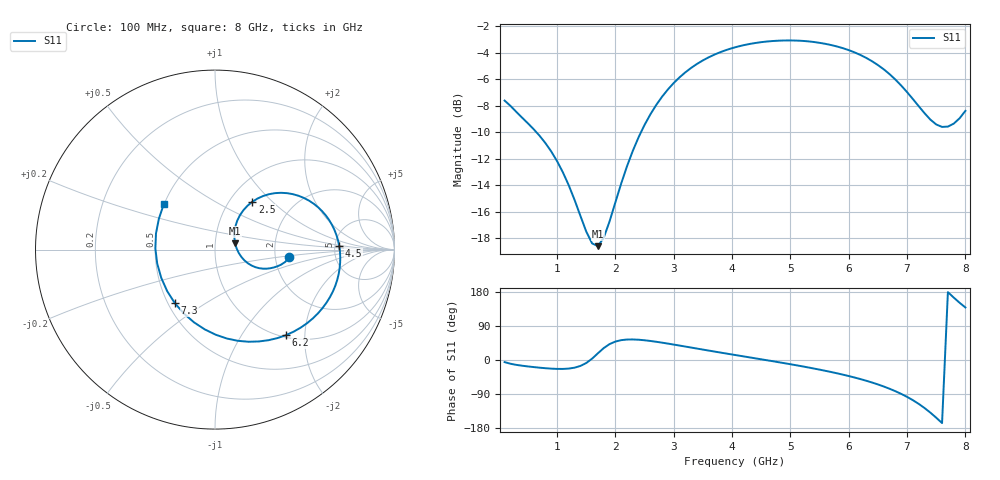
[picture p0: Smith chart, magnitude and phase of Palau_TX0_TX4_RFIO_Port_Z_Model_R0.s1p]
! Created Wed Jul  8 17:57:20 2020
! Palau TX0/TX4 RFIO Port Impedance Model.
! Revision		: R0.
! Impedance Mode 	: Balanced Differential-Mode.
! Impedance Format 	: Series Equivalent Differential Impedance (SEDZ).
# hz S ma R 50
! 1 Port Network Data from SP1.SP block
! freq  magS11  angS11
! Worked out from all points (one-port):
!   80 points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, 100 MHz to 8 GHz, reference 50 ohm
!   lowest |S11| = -18.6 dB at 1.7 GHz (marker M1), VSWR 1.27, Z = 62.4 + j4.54 ohm
!   |S11| at or under -10 dB: 645.5 MHz to 2.438 GHz (1.793 GHz wide, 116 % of centre)
!   S11 on the Smith chart (normalised r, x): 100 MHz: 2.40, -0.23; 2.5 GHz: 1.27, +0.76; 4.5 GHz: 5.45, +0.47; 6.2 GHz: 1.04, -1.61; 7.3 GHz: 0.54, -0.38; 8 GHz: 0.50, +0.29
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1e8  0.4164 -5.6
3e8  0.3777 -12.8
5e8  0.3417 -17.0
8e8  0.2877 -21.7
1.1e9  0.2231 -23.5
1.5e9  0.1334 -7.9
1.6e9  0.1204 3.6
1.7e9  0.1175 17.8
1.8e9  0.1265 31.5
2.1e9  0.2029 52.4
2.5e9  0.3373 52.1
2.8e9  0.4309 45.7
3.1e9  0.5099 38.1
3.6e9  0.6068 24.8
4.1e9  0.6661 12.0
4.5e9  0.6921 1.8
5.1e9  0.7016 -13.9
5.6e9  0.6819 -28.5
6.1e9  0.6332 -46.2
6.2e9  0.6192 -50.4
6.5e9  0.5672 -64.5
6.7e9  0.5241 -75.9
6.9e9  0.4745 -89.5
7.1e9  0.422 -106.0
7.3e9  0.3732 -126.8
7.5e9  0.3384 -152.3
7.7e9  0.3322 179.1
8e9  0.3809 138.6
